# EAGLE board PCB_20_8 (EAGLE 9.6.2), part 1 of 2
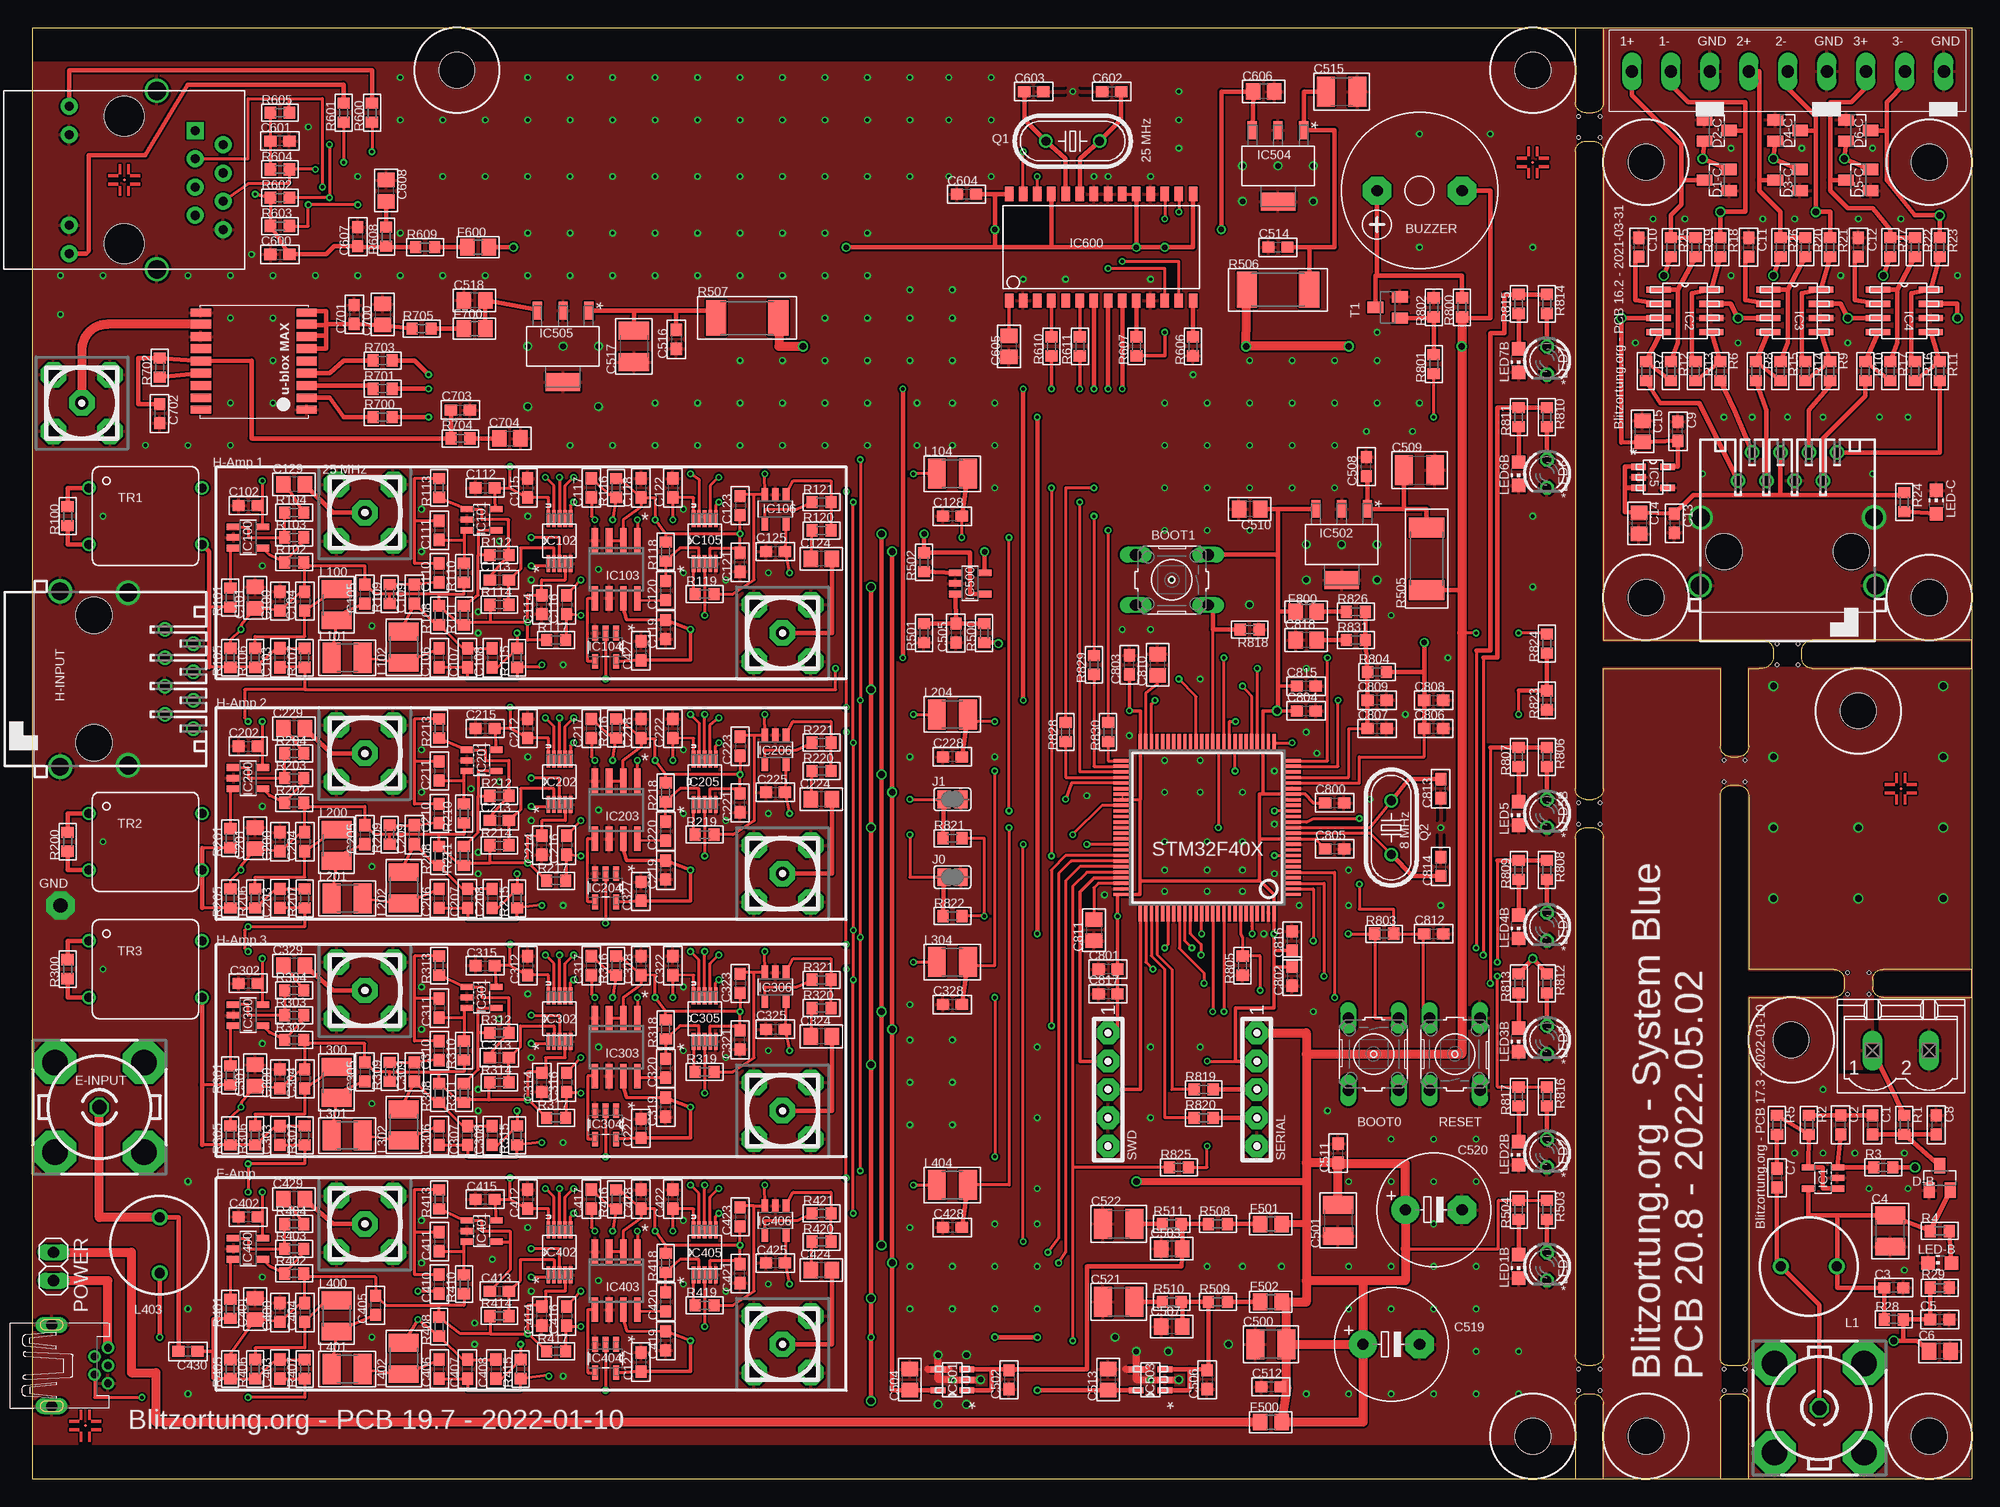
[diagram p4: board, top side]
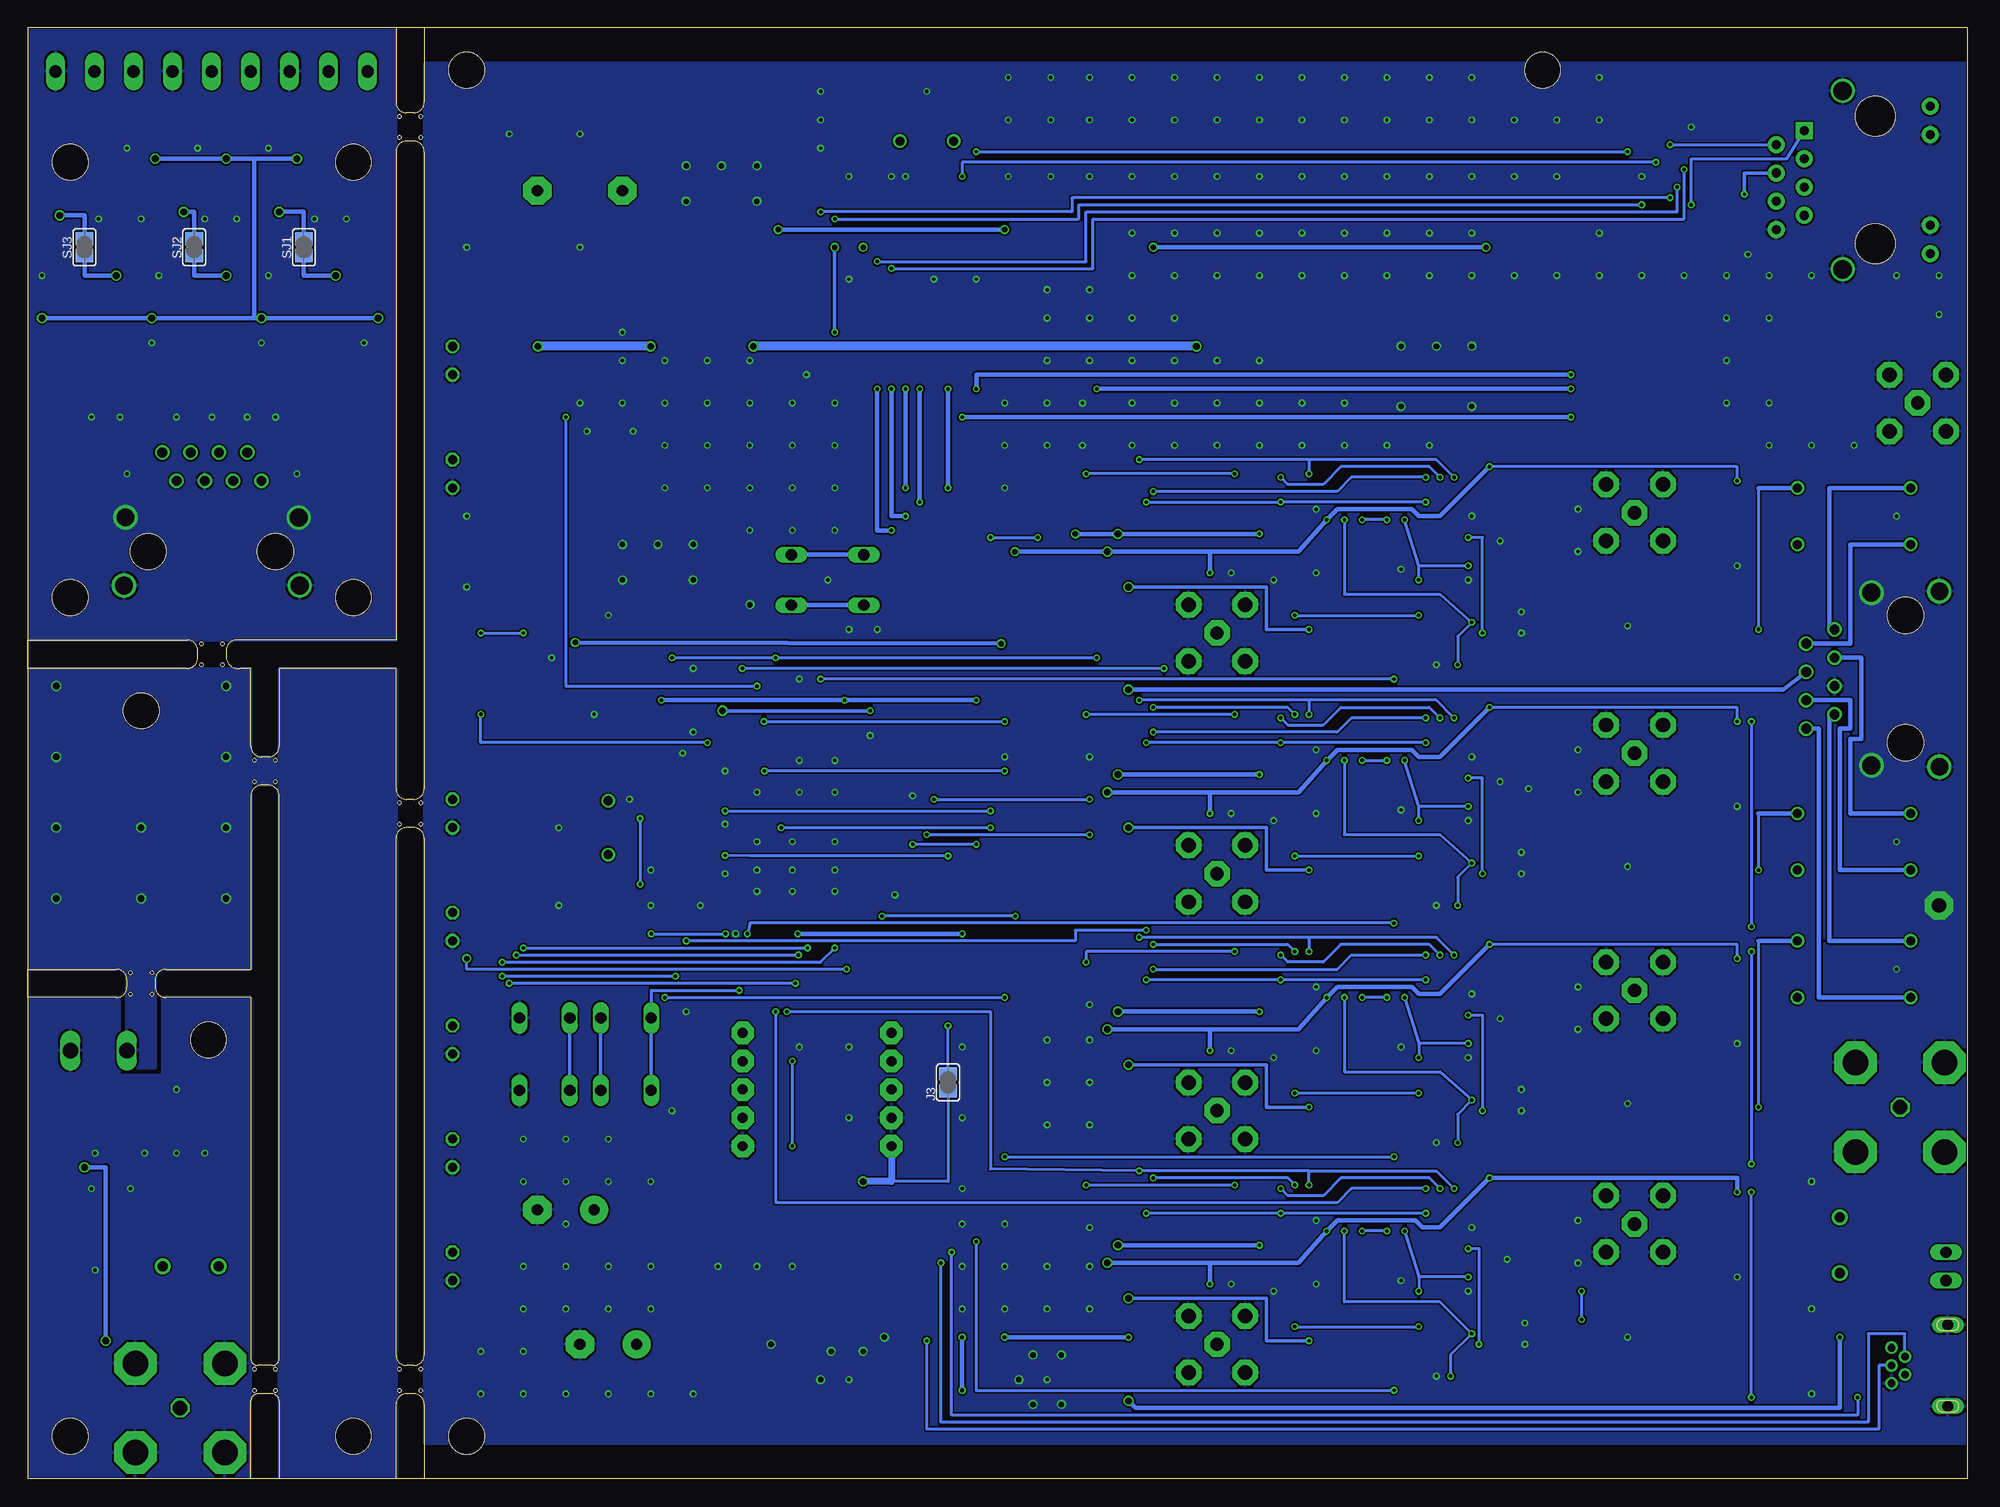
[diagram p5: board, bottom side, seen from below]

Size 173.99 x 130.18 mm. Coordinates in mm from the lower left corner, seen from the top.
Outline: 0,130.18 0,0 173.99,0 173.99,130.18 0,130.18
Copper layers (1*16): Top 0.035mm / dielectric 1.5mm / Bottom 0.035mm
Design rules "default *": minimum track width 6mil, minimum drill 12mil, track to track 6mil, track to pad 6mil, pad to pad 6mil, via to via 6mil, smd to smd 6mil, copper to edge 4mil, drill to drill 8mil, minimum pad ring 8mil, minimum via ring 6mil, stop-mask expansion 3mil, vias tented up to drill 12mil, thermal gap 8mil
Holes 3.2 mm at 134.62,126.36 134.62,3.81 38.1,126.36 157.8,39.37 170.18,3.81 170.18,79.06 144.78,79.06 170.18,118.11 144.78,118.11 163.83,68.9 144.78,3.81
Holes 0.3 mm at 156.53,74.93 158.43,74.93 158.43,73.03 156.53,73.03 138.75,60.64 138.75,58.74 140.65,58.74 140.65,60.64 162.88,43.5 164.78,43.5 164.78,45.4 162.88,45.4 138.75,9.84 138.75,7.94 140.65,7.94 140.65,9.84 151.76,9.84 151.76,7.94 153.67,7.94 153.67,9.84 138.75,122.24 138.75,120.33 140.65,120.33 140.65,122.24 153.67,64.45 151.76,64.45 151.76,62.55 153.67,62.55
tRestrict: 16 lines
Milling: 72 lines

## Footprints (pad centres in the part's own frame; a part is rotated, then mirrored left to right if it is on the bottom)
B3F-10XX = drill 1.016 long: 1 -3.251,2.261; 2 3.251,2.261; 3 -3.251,-2.261; 4 3.251,-2.261
F/CM12P = drill 1.016 pad 2.54 octagon: + 3.81,0; - -3.81,0
C0603 = smd 1.1 x 1: 1 -0.85,0; 2 0.85,0
C1210 = smd 1.6 x 2.7: 1 -1.4,0; 2 1.4,0
C0805 = smd 1.3 x 1.5: 1 -0.95,0; 2 0.95,0
E5-10,5 = drill 1.016 pad 2.54: + -2.54,0 | drill 1.016 pad 2.54 octagon: - 2.54,0
SOT23 = smd 1 x 1.4: 1 -0.95,-1.1; 2 0.95,-1.1; 3 0,1.1
R141426 = drill 1.3 octagon: 1 0,0 | drill 2.286 pad 3.81 octagon: 2 4.008,4.008; 3 -4.008,4.008; 4 -4.008,-4.008; 5 4.008,-4.008
R0805 = smd 1.3 x 1.5: 1 -0.95,0; 2 0.95,0
XLEMO02N = drill 1.3 pad 2.286 octagon: GND@1 -2.54,-2.54; GND@2 2.54,-2.54; GND@3 2.54,2.54; GND@4 -2.54,2.54 | drill 1.2 pad 2.286 octagon: SIG 0,0
556591-1 = drill 0.889: 1 -4.445,6.35; 2 -3.175,8.89; 3 -1.905,6.35; 4 -0.635,8.89; 5 0.635,6.35; 6 1.905,8.89; 7 3.175,6.35; 8 4.445,8.89 | drill 1.575 pad 2.184: G1 -7.874,-3.048; G2 7.874,-3.048 | hole 3.251: -5.715,0; 5.715,0
SOT23-5 = smd 0.55 x 1.2: 1 -0.95,-1.3; 2 0,-1.3; 3 0.95,-1.3; 4 0.95,1.3; 5 -0.95,1.3
SOIC127P600X175-8N = smd 2.184 x 0.559: 1 -2.362,1.905; 2 -2.362,0.635; 3 -2.362,-0.635; 4 -2.362,-1.905; 5 2.362,-1.905; 6 2.362,-0.635; 7 2.362,0.635; 8 2.362,1.905
SOT95P280X110-5N = smd 1.321 x 0.559: 1 -1.295,0.94; 2 -1.295,0; 3 -1.295,-0.94; 4 1.295,-0.94; 5 1.295,0.94
SOT23-5' = smd 0.6 x 1.2: 1 -0.95,-1.306; 2 0,-1.306; 3 0.95,-1.306; 4 0.95,1.306; 5 -0.95,1.306
SOP50P490X110-10N = smd 1.524 x 0.33: 1 -2.032,0.991; 2 -2.032,0.508; 3 -2.032,0; 4 -2.032,-0.508; 5 -2.032,-0.991; 6 2.032,-0.991; 7 2.032,-0.508; 8 2.032,0; 9 2.032,0.508; 10 2.032,0.991
SOIC8 = smd 0.6 x 2.2: 1 -1.905,-2.6; 2 -0.635,-2.6; 3 0.635,-2.6; 4 1.905,-2.6; 5 1.905,2.6; 6 0.635,2.6; 7 -0.635,2.6; 8 -1.905,2.6
SOT95P275X110-5N = smd 1.321 x 0.559: 1 -1.27,0.94; 2 -1.27,0; 3 -1.27,-0.94; 4 1.27,-0.94; 5 1.27,0.94
SOT230P696X180-4N = smd 1.6 x 0.838: 1 -3.2,2.311; 2 -3.2,0; 3 -3.2,-2.311 | smd 1.6 x 3.099: 4 3.2,0
SO28W = smd 0.762 x 1.27: 1 -7.62,-4.78; 2 -6.35,-4.78; 3 -5.08,-4.78; 4 -3.81,-4.78; 5 -2.54,-4.78; 6 -1.27,-4.78; 7 0,-4.78; 8 1.27,-4.78; 9 2.54,-4.78; 10 3.81,-4.78; 11 5.08,-4.78; 12 6.35,-4.78; 13 7.62,-4.78; 14 8.89,-4.78; 15 8.89,4.78; 16 7.62,4.78; 17 6.35,4.78; 18 5.08,4.78; 19 3.81,4.78; 20 2.54,4.78; 21 1.27,4.78; 22 0,4.78; 23 -1.27,4.78; 24 -2.54,4.78; 25 -3.81,4.78; 26 -5.08,4.78; 27 -6.35,4.78; 28 -7.62,4.78
LQFP100 = smd 1.6 x 0.3: 1 -7.6,6; 2 -7.6,5.5; 3 -7.6,5; 4 -7.6,4.5; 5 -7.6,4; 6 -7.6,3.5; 7 -7.6,3; 8 -7.6,2.5; 9 -7.6,2; 10 -7.6,1.5; 11 -7.6,1; 12 -7.6,0.5; 13 -7.6,0; 14 -7.6,-0.5; 15 -7.6,-1; 16 -7.6,-1.5; 17 -7.6,-2; 18 -7.6,-2.5; 19 -7.6,-3; 20 -7.6,-3.5; 21 -7.6,-4; 22 -7.6,-4.5; 23 -7.6,-5; 24 -7.6,-5.5; 25 -7.6,-6; 51 7.6,-6; 52 7.6,-5.5; 53 7.6,-5; 54 7.6,-4.5; 55 7.6,-4; 56 7.6,-3.5; 57 7.6,-3; 58 7.6,-2.5; 59 7.6,-2; 60 7.6,-1.5; 61 7.6,-1; 62 7.6,-0.5; 63 7.6,0; 64 7.6,0.5; 65 7.6,1; 66 7.6,1.5; 67 7.6,2; 68 7.6,2.5; 69 7.6,3; 70 7.6,3.5; 71 7.6,4; 72 7.6,4.5; 73 7.6,5; 74 7.6,5.5; 75 7.6,6 | smd 0.3 x 1.6: 26 -6,-7.6; 27 -5.5,-7.6; 28 -5,-7.6; 29 -4.5,-7.6; 30 -4,-7.6; 31 -3.5,-7.6; 32 -3,-7.6; 33 -2.5,-7.6; 34 -2,-7.6; 35 -1.5,-7.6; 36 -1,-7.6; 37 -0.5,-7.6; 38 0,-7.6; 39 0.5,-7.6; 40 1,-7.6; 41 1.5,-7.6; 42 2,-7.6; 43 2.5,-7.6; 44 3,-7.6; 45 3.5,-7.6; 46 4,-7.6; 47 4.5,-7.6; 48 5,-7.6; 49 5.5,-7.6; 50 6,-7.6; 76 6,7.6; 77 5.5,7.6; 78 5,7.6; 79 4.5,7.6; 80 4,7.6; 81 3.5,7.6; 82 3,7.6; 83 2.5,7.6; 84 2,7.6; 85 1.5,7.6; 86 1,7.6; 87 0.5,7.6; 88 0,7.6; 89 -0.5,7.6; 90 -1,7.6; 91 -1.5,7.6; 92 -2,7.6; 93 -2.5,7.6; 94 -3,7.6; 95 -3.5,7.6; 96 -4,7.6; 97 -4.5,7.6; 98 -5,7.6; 99 -5.5,7.6; 100 -6,7.6
MSTBV2 = drill 1.397 long: 1 -2.54,0; 2 2.54,0
SJ = smd 1.168 x 1.6: 1 -0.762,0; 2 0.762,0
6000-XXXX-RC = drill 0.9 pad 1.422: 1 -2.5,0; 2 2.5,0
R1210 = smd 1.6 x 2.7: 1 -1.4,0; 2 1.4,0
LED3MM = drill 0.813 octagon: A -1.27,0; K 1.27,0
CHIP-LED0805 = smd 1.2 x 1.2: A 0,-1.05; C 0,1.05
PASSER-SMD = smd 0.254 x 0.254: PASS@1 0,0
1X02 = drill 1.016 long: 1 -1.27,0; 2 1.27,0
HC49U-V = drill 0.813: 1 -2.413,0; 2 2.413,0
R0603 = smd 1 x 1.1: 1 -0.85,0; 2 0.85,0
R2512 = smd 1.8 x 3.2: 1 -2.8,0; 2 2.8,0
HR911105A = drill 0.813 pad 1.524: G+ 4.953,-6.604; G- 4.953,-4.064; GND -8.89,4.445; NC -6.35,3.175; P4 -8.89,-0.635; P5 -6.35,0.635; RD+ -6.35,-1.905; RD- -8.89,1.905; TD- -8.89,-3.175; Y+ 4.953,6.604; Y- 4.953,4.064 | drill 1.651 pad 2.159: SHIELD0 -2.921,8.001; SHIELD1 -2.921,-8.001 | drill 0.813 pad 1.524 square: TD+ -6.35,-4.445 | hole 3.556: 0,-5.715; 0,5.715
X05N-SIL = drill 0.889 pad 2.032 octagon: 1 -5.08,0; 2 -2.54,0; 3 0,0; 4 2.54,0; 5 5.08,0
786-4 = drill 0.8: 1 -5.08,2.54; 3 -5.08,-2.54; 4 5.08,-2.54; 6 5.08,2.54
MAX-M8 = smd 1.8 x 0.7: 1_GND 4.95,-4.4; 9_RESET_N 4.95,4.3; 10_GND -4.55,4.3; 18_SAFEBOOT_N -4.55,-4.4 | smd 1.8 x 0.8: 2_TXD 4.95,-3.35; 3_RXD 4.95,-2.25; 4_TIMEPULSE 4.95,-1.15; 5_EXTINT 4.95,-0.05; 6_V_BCKP 4.95,1.05; 7_VCC_IO 4.95,2.15; 8_VCC 4.95,3.25; 11_RF_IN -4.55,3.25; 12_GND -4.55,2.15; 13_LNA_EN -4.55,1.05; 14_VCC_RF -4.55,-0.05; 15_V_ANT/RESERVED -4.55,-1.15; 16_SDA -4.55,-2.25; 17_SCL -4.55,-3.35
32005-601 = drill 0.7 pad 1.016: 1 2.825,1.6; 2 1.625,0.8; 3 2.825,0; 4 1.625,-0.8; 5 2.825,-1.6 | drill 1 pad 1.422 long: M1 -2.225,3.65; M2 -2.225,-3.65
1751316 = drill 1.1 pad 1.7 long: 1 -13.973,-0.1; 2 -10.473,-0.1; 3 -6.973,-0.1; 4 -3.473,-0.1; 5 0.028,-0.1; 6 3.527,-0.1; 7 7.027,-0.1; 8 10.527,-0.1; 9 14.027,-0.1

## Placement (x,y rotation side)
BOOT0  boot0  [B3F-10XX]  120.33,38.1 270 top
BOOT1  boot1  [B3F-10XX]  102.23,80.64 180 top
BUZZER  F/CM12P  [F/CM12P]  124.46,115.57 180 top
C1  10pF  [C0603]  165.1,31.75 270 top
C2  10pF  [C0603]  162.24,31.75 90 top
C3  1uF  [C0603]  167,17.14 180 top
C4  47uF  [C1210]  166.69,22.23 90 top
C5  1uF  [C0603]  171.13,14.29 180 top
C6  10uF  [C0805]  171.13,11.43 180 top
C7  1uF  [C0603]  156.53,26.99 90 top
C8  47pF  [C0603]  170.81,31.75 270 top
C9  100nF  [C0603]  147.64,93.98 90 top
C10  100nF  [C0603]  144.15,110.49 90 top
C11  100nF  [C0603]  153.99,110.49 90 top
C12  100nF  [C0603]  163.83,110.49 90 top
C13  100nF  [C0603]  147.32,85.72 270 top
C14  10uF  [C0805]  144.15,85.72 270 top
C15  10uF  [C0805]  144.46,93.98 90 top
C100  1uF  [C0603]  22.23,78.74 270 top
C101  10uF  [C0805]  20,79.06 270 top
C102  1uF  [C0603]  19.37,87.31 0 top
C103  4.7pF  [C0603]  22.23,73.66 90 top
C104  1.5nF  [C0603]  24.45,78.74 270 top
C105  6.8nF  [C0603]  29.84,79.38 270 top
C106  12nF  [C0603]  36.51,73.66 90 top
C107  22nF  [C0603]  39.05,73.66 90 top
C108  2.2nF  [C0603]  41.27,73.66 270 top
C109  1nF  [C0603]  34.29,79.38 90 top
C110  1nF  [C0603]  36.51,81.28 90 top
C111  1nF  [C0603]  36.51,85.09 270 top
C112  1uF  [C0603]  40.64,88.9 0 top
C113  1uF  [C0603]  41.91,80.64 0 top
C114  1uF  [C0603]  45.72,78.42 90 top
C115  1uF  [C0603]  44.45,88.9 270 top
C116  1uF  [C0603]  47.94,78.42 270 top
C117  1uF  [C0603]  50.16,88.9 90 top
C118  1uF  [C0603]  54.61,88.9 270 top
C119  1uF  [C0603]  56.83,76.2 90 top
C120  1uF  [C0603]  56.83,79.69 90 top
C121  1uF  [C0603]  63.5,82.23 90 top
C122  1uF  [C0603]  57.47,88.9 270 top
C123  750pF  [C0603]  63.5,87.31 270 top
C124  10uF  [C0805]  70.8,82.55 180 top
C125  1uF  [C0603]  66.67,83.19 0 top
C127  100nF  [C0603]  54.61,10.48 270 top
C128  3.3nF  [C0603]  82.55,86.36 180 top
C129  10uF  [C0805]  23.5,89.22 180 top
C200  1uF  [C0603]  22.23,57.15 270 top
C201  10uF  [C0805]  20,57.47 270 top
C202  1uF  [C0603]  19.37,65.72 0 top
C203  4.7pF  [C0603]  22.23,52.07 90 top
C204  1.5nF  [C0603]  24.45,57.15 270 top
C205  6.8nF  [C0603]  29.84,57.78 270 top
C206  12nF  [C0603]  36.51,52.07 90 top
C207  22nF  [C0603]  39.05,52.07 90 top
C208  2.2nF  [C0603]  41.27,52.07 270 top
C209  1nF  [C0603]  34.29,57.78 90 top
C210  1nF  [C0603]  36.51,59.69 90 top
C211  1nF  [C0603]  36.51,63.5 270 top
C212  1uF  [C0603]  44.45,67.31 270 top
C213  1uF  [C0603]  41.91,59.05 0 top
C214  1uF  [C0603]  45.72,56.83 90 top
C215  1uF  [C0603]  40.64,67.31 0 top
C216  1uF  [C0603]  47.94,56.83 270 top
C217  1uF  [C0603]  50.16,67.31 90 top
C218  1uF  [C0603]  54.61,67.31 270 top
C219  1uF  [C0603]  56.83,54.61 90 top
C220  1uF  [C0603]  56.83,58.1 90 top
C221  1uF  [C0603]  63.5,60.64 90 top
C222  1uF  [C0603]  57.47,67.31 270 top
C223  750pF  [C0603]  63.5,65.72 270 top
C224  10uF  [C0805]  70.8,60.96 180 top
C225  1uF  [C0603]  66.67,61.59 0 top
C227  100nF  [C0603]  54.61,31.43 270 top
C228  3.3nF  [C0603]  82.55,64.77 180 top
C229  10uF  [C0805]  23.5,67.31 180 top
C300  1uF  [C0603]  22.23,35.88 270 top
C301  10uF  [C0805]  20,36.2 270 top
C302  1uF  [C0603]  19.37,44.45 0 top
C303  4.7pF  [C0603]  22.23,30.8 90 top
C304  1.5nF  [C0603]  24.45,35.88 270 top
C305  6.8nF  [C0603]  29.84,36.51 270 top
C306  12nF  [C0603]  36.51,30.8 90 top
C307  22nF  [C0603]  39.05,30.8 90 top
C308  2.2nF  [C0603]  41.27,30.8 270 top
C309  1nF  [C0603]  34.29,36.51 90 top
C310  1nF  [C0603]  36.51,38.42 90 top
C311  1nF  [C0603]  36.51,42.23 270 top
C312  1uF  [C0603]  44.45,46.04 270 top
C313  1uF  [C0603]  41.91,37.78 0 top
C314  1uF  [C0603]  45.72,35.56 90 top
C315  1uF  [C0603]  40.64,46.04 0 top
C316  1uF  [C0603]  47.94,35.56 270 top
C317  1uF  [C0603]  50.16,46.04 90 top
C318  1uF  [C0603]  54.61,46.04 270 top
C319  1uF  [C0603]  56.83,33.34 90 top
C320  1uF  [C0603]  56.83,36.83 90 top
C321  1uF  [C0603]  63.5,39.37 90 top
C322  1uF  [C0603]  57.47,46.04 270 top
C323  750pF  [C0603]  63.5,44.45 270 top
C324  10uF  [C0805]  70.8,39.69 180 top
C325  1uF  [C0603]  66.67,40.32 0 top
C327  100nF  [C0603]  54.61,52.7 270 top
C328  3.3nF  [C0603]  82.55,42.55 180 top
C329  10uF  [C0805]  23.5,46.04 180 top
C400  1uF  [C0603]  22.23,14.92 270 top
C401  10uF  [C0805]  20,15.24 270 top
C402  1uF  [C0603]  19.37,23.5 0 top
C403  4.7pF  [C0603]  22.23,9.84 90 top
C404  1.5nF  [C0603]  24.45,14.92 270 top
C405  6.8nF  [C0603]  30.8,15.56 270 top
C406  12nF  [C0603]  36.51,9.84 90 top
C407  22nF  [C0603]  39.05,9.84 90 top
C408  2.2nF  [C0603]  41.59,9.84 270 top
C410  1nF  [C0603]  36.51,17.46 90 top
C411  1nF  [C0603]  36.51,21.27 270 top
C412  1uF  [C0603]  44.45,25.08 270 top
C413  1uF  [C0603]  41.91,16.83 0 top
C414  1uF  [C0603]  45.72,14.61 90 top
C415  1uF  [C0603]  40.64,25.08 0 top
C416  1uF  [C0603]  47.94,14.61 270 top
C417  1uF  [C0603]  50.16,25.08 90 top
C418  1uF  [C0603]  54.61,25.08 270 top
C419  1uF  [C0603]  56.83,12.38 90 top
C420  1uF  [C0603]  56.83,15.88 90 top
C421  1uF  [C0603]  63.5,18.41 90 top
C422  1uF  [C0603]  57.47,25.08 270 top
C423  750pF  [C0603]  63.5,23.5 270 top
C424  10uF  [C0805]  70.8,18.73 180 top
C425  1uF  [C0603]  66.67,19.37 0 top
C427  100nF  [C0603]  54.61,74.3 270 top
C428  3.3nF  [C0603]  82.55,22.54 180 top
C429  10uF  [C0805]  23.5,25.08 180 top
C430  1uF  [C0603]  13.97,11.43 0 top
C500  47uF  [C1210]  111.12,12.06 180 top
C501  47uF  [C1210]  117.16,23.18 270 top
C502  100nF  [C0603]  87.63,8.89 270 top
C503  10uF  [C0805]  102.23,20.64 180 top
C504  10uF  [C0805]  78.74,8.89 90 top
C505  1uF  [C0603]  82.87,75.88 270 top
C506  100nF  [C0603]  105.41,8.89 270 top
C507  10uF  [C0805]  102.23,13.65 180 top
C508  100nF  [C0603]  119.7,90.81 90 top
C509  47uF  [C1210]  124.46,90.49 0 top
C510  10uF  [C0805]  109.22,87 180 top
C511  100nF  [C0603]  117.16,29.21 90 top
C512  100nF  [C0603]  111.12,8.26 180 top
C513  10uF  [C0805]  96.52,8.89 90 top
C514  100nF  [C0603]  111.76,110.49 180 top
C515  47uF  [C1210]  117.47,124.46 0 top
C516  100nF  [C0603]  57.78,102.23 270 top
C517  47uF  [C1210]  53.98,101.6 270 top
C518  10uF  [C0805]  39.69,105.73 180 top
C519  1000uF  [E5-10,5]  121.92,12.06 0 top
C520  1000uF  [E5-10,5]  125.73,24.13 0 top
C521  47uF  [C1210]  97.47,15.88 0 top
C522  47uF  [C1210]  97.47,22.86 0 top
C600  100nF  [C0603]  22.23,109.86 0 top
C601  100nF  [C0603]  22.23,120.02 180 top
C602  18pF  [C0603]  96.84,124.46 0 top
C603  18pF  [C0603]  89.85,124.46 180 top
C604  100nF  [C0603]  83.82,115.25 0 top
C605  10uF  [C0805]  87.63,101.6 90 top
C606  10uF  [C0805]  110.49,124.46 180 top
C607  1uF  [C0603]  29.21,111.44 90 top
C608  10uF  [C0805]  31.75,115.57 90 top
C700  10uF  [C0805]  31.43,104.46 270 top
C701  100nF  [C0603]  28.89,104.46 270 top
C702  100nF  [C0603]  11.43,95.57 270 top
C703  1uF  [C0603]  38.42,95.89 0 top
C704  10uF  [C0805]  42.86,93.34 0 top
C800  100nF  [C0603]  116.84,60.64 0 top
C801  100nF  [C0603]  96.52,45.72 180 top
C802  100nF  [C0603]  113.03,45.09 270 top
C803  100nF  [C0603]  98.42,73.03 90 top
C804  100nF  [C0603]  114.3,68.9 0 top
C805  100nF  [C0603]  116.84,56.52 0 top
C806  1uF  [C0603]  125.73,67.31 0 top
C807  1uF  [C0603]  120.65,67.31 180 top
C808  100nF  [C0603]  125.73,69.85 0 top
C809  100nF  [C0603]  120.65,69.85 180 top
C810  10uF  [C0805]  100.97,73.03 90 top
C811  10uF  [C0805]  95.25,49.21 270 top
C812  100nF  [C0603]  125.73,48.9 0 top
C813  18pF  [C0603]  126.36,61.91 90 top
C814  18pF  [C0603]  126.36,54.93 270 top
C815  1uF  [C0603]  114.3,71.12 0 top
C816  1uF  [C0603]  113.03,48.26 90 top
C817  1uF  [C0603]  96.52,43.5 180 top
C818  10uF  [C0805]  114.3,75.25 180 top
D1-C  BAT54S  [SOT23]  151.13,116.52 90 top
D2-C  BAT54S  [SOT23]  151.13,120.97 270 top
D3-C  BAT54S  [SOT23]  157.48,116.52 90 top
D4-C  BAT54S  [SOT23]  157.48,120.97 270 top
D5-C  BAT54S  [SOT23]  163.83,116.52 90 top
D6-C  BAT54S  [SOT23]  163.83,120.97 270 top
D-B  BAT54S  [SOT23]  171.13,26.99 0 top
E-INPUT  [R141426]  6.03,33.34 0 top
F500  60  [R0805]  111.12,5.08 180 top
F501  220  [R0805]  111.12,22.86 180 top
F502  220  [R0805]  111.12,15.88 180 top
F600  60  [R0805]  40.01,110.49 180 top
F700  60  [R0805]  39.69,103.19 180 top
F800  220  [R0805]  114.3,77.79 180 top
GPS-IN  GPS-IN  [XLEMO02N]  4.45,96.52 0 top
H-INPUT  RJ45  [556591-1]  5.56,71.75 270 top
IC1  ADA4891  [SOT23-5]  160.66,26.99 90 top
IC2  THS4531ID  [SOIC127P600X175-8N]  148.27,104.78 0 top
IC3  THS4531ID  [SOIC127P600X175-8N]  158.12,104.78 0 top
IC4  THS4531ID  [SOIC127P600X175-8N]  167.96,104.78 0 top
IC5  TLV70033  [SOT95P280X110-5N]  145.41,89.85 0 top
IC100  MCP6021  [SOT23-5']  19.37,84.45 270 top
IC101  ADA4891  [SOT23-5]  40.32,86.04 270 top
IC102  MCP6S93-E/UN  [SOP50P490X110-10N]  47.31,84.14 90 top
IC103  LTC1569CS8-7  [SOIC8]  52.39,81.6 180 top
IC104  MC74HC1G04DTT1G  [SOT95P275X110-5N]  51.44,74.61 270 top
IC105  MCP6S93-E/UN  [SOP50P490X110-10N]  60.33,84.14 90 top
IC106  MCP6021  [SOT23-5']  66.67,87 180 top
IC200  MCP6021  [SOT23-5']  19.37,62.87 270 top
IC201  ADA4891  [SOT23-5]  40.32,64.45 270 top
IC202  MCP6S93-E/UN  [SOP50P490X110-10N]  47.31,62.55 90 top
IC203  LTC1569CS8-7  [SOIC8]  52.39,60.01 180 top
IC204  MC74HC1G04DTT1G  [SOT95P275X110-5N]  51.44,53.02 270 top
IC205  MCP6S93-E/UN  [SOP50P490X110-10N]  60.33,62.55 90 top
IC206  MCP6021  [SOT23-5']  66.67,65.41 180 top
IC300  MCP6021  [SOT23-5']  19.37,41.59 270 top
IC301  ADA4891  [SOT23-5]  40.32,43.18 270 top
IC302  MCP6S93-E/UN  [SOP50P490X110-10N]  47.31,41.27 90 top
IC303  LTC1569CS8-7  [SOIC8]  52.39,38.73 180 top
IC304  MC74HC1G04DTT1G  [SOT95P275X110-5N]  51.44,31.75 270 top
IC305  MCP6S93-E/UN  [SOP50P490X110-10N]  60.33,41.27 90 top
IC306  MCP6021  [SOT23-5']  66.67,44.13 180 top
IC400  MCP6021  [SOT23-5']  19.37,20.64 270 top
IC401  ADA4891  [SOT23-5]  40.32,22.23 270 top
IC402  MCP6S93-E/UN  [SOP50P490X110-10N]  47.31,20.32 90 top
IC403  LTC1569CS8-7  [SOIC8]  52.39,17.78 180 top
IC404  MC74HC1G04DTT1G  [SOT95P275X110-5N]  51.44,10.79 270 top
IC405  MCP6S93-E/UN  [SOP50P490X110-10N]  60.33,20.32 90 top
IC406  MCP6021  [SOT23-5']  66.67,23.18 180 top
IC500  ADA4891  [SOT23-5']  84.14,80.33 270 top
IC501  TLV70033  [SOT95P280X110-5N]  82.55,8.89 180 top
IC502  LM3940IMP-3.3  [SOT230P696X180-4N]  117.47,83.82 270 top
IC503  LP5907MFX-4.5NPB  [SOT95P280X110-5N]  100.33,8.89 180 top
IC504  LM3940IMP-3.3  [SOT230P696X180-4N]  111.76,117.79 270 top
IC505  LM3940IMP-3.3  [SOT230P696X180-4N]  47.62,101.6 270 top
IC600  ENC28J60SO  [SO28W]  95.25,110.49 0 top
IC800  STM32D40X  [LQFP100]  105.41,58.42 180 top
IN  MSTBV2  [MSTBV2]  167.64,38.42 0 top
J0  J0  [SJ]  82.55,53.98 0 top
J1  J1  [SJ]  82.55,60.96 0 top
J2  Amplifier  [556591-1]  157.48,83.19 0 top
J3  J1  [SJ]  91.44,35.56 90 bottom
L1  3.3mH  [6000-XXXX-RC]  159.38,19.05 180 top
L100  330uH  [R1210]  27.3,78.42 270 top
L101  680uH  [R1210]  28.26,73.66 0 top
L102  1mH  [R1210]  33.34,74.61 90 top
L104  22uH  [R1210]  82.55,90.17 180 top
L200  330uH  [R1210]  27.3,56.83 270 top
L201  680uH  [R1210]  28.26,52.07 0 top
L202  1mH  [R1210]  33.34,53.02 90 top
L204  22uH  [R1210]  82.55,68.58 180 top
L300  330uH  [R1210]  27.3,35.56 270 top
L301  680uH  [R1210]  28.26,30.8 0 top
L302  1mH  [R1210]  33.34,31.75 90 top
L304  22uH  [R1210]  82.55,46.35 180 top
L400  330uH  [R1210]  27.3,14.61 270 top
L401  680uH  [R1210]  28.26,9.84 0 top
L402  1mH  [R1210]  33.34,10.79 90 top
L403  3.3mH  [6000-XXXX-RC]  11.43,20.95 90 top
L404  22uH  [R1210]  82.55,26.35 180 top
LED1  Power  [LED3MM]  135.89,19.05 270 top
LED1B  Power  [CHIP-LED0805]  133.35,19.05 180 top
LED2  Mode  [LED3MM]  135.89,29.21 270 top
LED2B  Mode  [CHIP-LED0805]  133.35,29.21 180 top
LED3  Network  [LED3MM]  135.89,39.37 270 top
LED3B  Network  [CHIP-LED0805]  133.35,39.37 180 top
LED4  Fault  [LED3MM]  135.89,49.53 270 top
LED4B  Fault  [CHIP-LED0805]  133.35,49.53 180 top
LED5  GPS  [LED3MM]  135.89,59.69 270 top
LED5B  GPS  [CHIP-LED0805]  133.35,59.69 180 top
LED6  Alarm  [LED3MM]  135.89,90.17 270 top
LED6B  Alarm  [CHIP-LED0805]  133.35,90.17 180 top
LED7  Signal  [LED3MM]  135.89,100.33 270 top
LED7B  Signal  [CHIP-LED0805]  133.35,100.33 180 top
LED-B  LED-B  [CHIP-LED0805]  171.13,19.37 90 top
LED-C  LED-C  [CHIP-LED0805]  170.81,87.63 0 top
OUT  R141426  [R141426]  160.34,6.35 270 top
PASSER1  [PASSER-SMD]  4.76,4.76 0 top
PASSER2  [PASSER-SMD]  8.26,116.52 0 top
PASSER3  [PASSER-SMD]  134.62,118.11 0 top
PASSER4  [PASSER-SMD]  167.64,61.91 0 top
POWER  power  [1X02]  1.91,19.05 270 top
Q1  25MHz  [HC49U-V]  93.34,120.02 0 top
Q2  8MHz  [HC49U-V]  121.92,58.42 90 top
R1  10K  [R0603]  167.96,31.75 90 top
R2  5.6M  [R0603]  159.38,31.75 90 top
R3  10M  [R0603]  166.05,27.94 180 top
R4  2.2K  [R0603]  171.13,22.23 180 top
R5  75  [R0603]  156.53,31.75 270 top
R6  49.9  [R0603]  151.45,99.38 270 top
R7  49.9  [R0603]  144.78,99.38 270 top
R8  49.9  [R0603]  154.62,99.38 270 top
R9  49.9  [R0603]  161.29,99.38 270 top
R10  49.9  [R0603]  164.47,99.38 270 top
R11  49.9  [R0603]  171.13,99.38 270 top
R12  10K  [R0603]  147,99.38 90 top
R13  10K  [R0603]  149.22,99.38 90 top
R14  10K  [R0603]  159.07,99.38 90 top
R15  10K  [R0603]  156.84,99.38 90 top
R16  10K  [R0603]  168.91,99.38 90 top
R17  10K  [R0603]  166.69,99.38 90 top
R18  1K  [R0603]  151.45,110.49 90 top
R19  1K  [R0603]  149.22,110.49 90 top
R20  1K  [R0603]  159.07,110.49 90 top
R21  1K  [R0603]  161.29,110.49 90 top
R22  1K  [R0603]  168.91,110.49 90 top
R23  1K  [R0603]  171.13,110.49 90 top
R24  2.2K  [R0603]  167.96,87.63 270 top
R25  160  [R0603]  147,110.49 270 top
R26  160  [R0603]  156.84,110.49 270 top
R27  160  [R0603]  166.69,110.49 270 top
R28  100K  [R0603]  167,14.29 180 top
R29  100K  [R0603]  171.13,17.14 180 top
R100  160  [R0603]  3.17,86.36 90 top
R101  1K  [R0603]  17.78,79.06 90 top
R102  1K  [R0603]  23.5,82.23 0 top
R103  1K  [R0603]  23.5,84.45 0 top
R104  49.9  [R0603]  23.5,86.68 0 top
R105  330  [R0603]  17.78,73.66 270 top
R106  270  [R0603]  20,73.66 90 top
R107  47K  [R0603]  24.45,73.66 270 top
R108  2.2K  [R0603]  36.51,77.47 270 top
R109  51K  [R0603]  32.07,79.38 90 top
R110  100K  [R0603]  38.73,81.28 90 top
R111  10K  [R0603]  38.73,77.47 90 top
R112  30K  [R0603]  41.91,82.87 0 top
R113  200K  [R0603]  36.51,88.9 270 top
R114  10K  [R0603]  41.91,78.42 0 top
R115  22K  [R0603]  43.5,73.66 90 top
R116  10K  [R0603]  52.39,88.9 270 top
R117  10K  [R0603]  46.99,75.25 0 top
R118  10K  [R0603]  56.83,83.19 270 top
R119  100  [R0603]  60.33,79.38 0 top
R120  49.9  [R0603]  70.8,85.09 180 top
R121  1K  [R0603]  70.8,87.63 0 top
R200  160  [R0603]  3.17,57.15 90 top
R201  1K  [R0603]  17.78,57.47 90 top
R202  1K  [R0603]  23.5,60.64 0 top
R203  1K  [R0603]  23.5,62.87 0 top
R204  49.9  [R0603]  23.5,65.09 0 top
R205  330  [R0603]  17.78,52.07 270 top
R206  270  [R0603]  20,52.07 90 top
R207  47K  [R0603]  24.45,52.07 270 top
R208  2.2K  [R0603]  36.51,55.88 270 top
R209  51K  [R0603]  32.07,57.78 90 top
R210  100K  [R0603]  38.73,59.69 90 top
R211  10K  [R0603]  38.73,55.88 90 top
R212  30K  [R0603]  41.91,61.28 0 top
R213  200K  [R0603]  36.51,67.31 270 top
R214  10K  [R0603]  41.91,56.83 0 top
R215  22K  [R0603]  43.5,52.07 90 top
R216  10K  [R0603]  52.39,67.31 270 top
R217  10K  [R0603]  46.99,53.66 0 top
R218  10K  [R0603]  56.83,61.59 270 top
R219  100  [R0603]  60.33,57.78 0 top
R220  49.9  [R0603]  70.8,63.5 180 top
R221  1K  [R0603]  70.8,66.04 0 top
R300  160  [R0603]  3.17,45.72 90 top
R301  1K  [R0603]  17.78,36.2 90 top
R302  1K  [R0603]  23.5,39.37 0 top
R303  1K  [R0603]  23.5,41.59 0 top
R304  49.9  [R0603]  23.5,43.81 0 top
R305  330  [R0603]  17.78,30.8 270 top
R306  270  [R0603]  20,30.8 90 top
R307  47K  [R0603]  24.45,30.8 270 top
R308  2.2K  [R0603]  36.51,34.61 270 top
R309  51K  [R0603]  32.07,36.51 90 top
R310  100K  [R0603]  38.73,38.42 90 top
R311  10K  [R0603]  38.73,34.61 90 top
R312  30K  [R0603]  41.91,40.01 0 top
R313  200K  [R0603]  36.51,46.04 270 top
R314  10K  [R0603]  41.91,35.56 0 top
R315  22K  [R0603]  43.5,30.8 90 top
R316  10K  [R0603]  52.39,46.04 270 top
R317  10K  [R0603]  46.99,32.38 0 top
R318  10K  [R0603]  56.83,40.32 270 top
R319  100  [R0603]  60.33,36.51 0 top
R320  49.9  [R0603]  70.8,42.23 180 top
R321  1K  [R0603]  70.8,44.77 0 top
R401  1K  [R0603]  17.78,15.24 90 top
R402  1K  [R0603]  23.5,18.41 0 top
R403  1K  [R0603]  23.5,20.64 0 top
R404  49.9  [R0603]  23.5,22.86 0 top
R405  82  [R0603]  17.78,9.84 90 top
R406  270  [R0603]  20,9.84 90 top
R407  47K  [R0603]  24.45,9.84 270 top
R408  2.2K  [R0603]  36.51,13.65 90 top
R410  150K  [R0603]  38.73,17.46 90 top
R413  68K  [R0603]  36.51,25.08 270 top
R414  10K  [R0603]  41.91,14.61 0 top
R415  22K  [R0603]  43.81,9.84 90 top
R416  10K  [R0603]  52.39,25.08 270 top
R417  10K  [R0603]  46.99,11.43 0 top
R418  10K  [R0603]  56.83,19.37 270 top
R419  100  [R0603]  60.33,15.56 0 top
R420  49.9  [R0603]  70.8,21.27 180 top
R421  1K  [R0603]  70.8,23.81 0 top
R500  1M  [R0603]  85.41,75.88 90 top
R501  1M  [R0603]  80.01,75.88 270 top
R502  10  [R0603]  80.01,82.23 270 top
R503  1K  [R0603]  135.89,24.13 90 top
R504  2.2K  [R0603]  133.35,24.13 90 top
R505  1.5  [R2512]  125.09,82.55 90 top
R506  1.5  [R2512]  111.76,106.68 0 top
R507  1.5  [R2512]  64.14,104.14 180 top
R508  0.27  [R0603]  106.36,22.86 180 top
R509  0.27  [R0603]  106.36,15.88 180 top
R510  0.27  [R0603]  102.23,15.88 0 top
R511  0.27  [R0603]  102.23,22.86 0 top
R600  680  [R0603]  30.48,122.56 90 top
R601  680  [R0603]  27.94,122.56 90 top
R602  49.9  [R0603]  22.23,114.94 180 top
R603  49.9  [R0603]  22.23,112.39 180 top
R604  49.9  [R0603]  22.23,117.47 0 top
R605  49.9  [R0603]  22.23,122.56 0 top
R606  2.2K  [R0603]  104.14,101.6 90 top
R607  10K  [R0603]  99.06,101.6 270 top
R608  0.27  [R0603]  31.75,111.44 270 top
R609  0.27  [R0603]  35.24,110.49 180 top
R610  75  [R0603]  91.44,101.6 270 top
R611  75  [R0603]  93.98,101.6 270 top
R700  470  [R0603]  31.43,95.25 180 top
R701  470  [R0603]  31.43,97.79 180 top
R702  10  [R0603]  11.43,99.69 90 top
R703  100  [R0603]  31.43,100.33 180 top
R704  0.27  [R0603]  38.42,93.34 180 top
R705  0.27  [R0603]  34.92,103.19 180 top
R800  470  [R0603]  128.27,105.09 270 top
R801  2.2K  [R0603]  125.73,100.01 270 top
R802  2.2K  [R0603]  125.73,105.09 270 top
R803  2.2K  [R0603]  121.28,48.9 180 top
R804  5.1  [R0603]  120.65,72.39 0 top
R805  10K  [R0603]  108.58,46.04 90 top
R806  4.7K  [R0603]  135.89,64.77 90 top
R807  1K  [R0603]  133.35,64.77 90 top
R808  330  [R0603]  135.89,54.61 90 top
R809  1K  [R0603]  133.35,54.61 90 top
R810  330  [R0603]  135.89,95.25 90 top
R811  1K  [R0603]  133.35,95.25 90 top
R812  330  [R0603]  135.89,44.45 90 top
R813  1K  [R0603]  133.35,44.45 90 top
R814  330  [R0603]  135.89,105.41 90 top
R815  1K  [R0603]  133.35,105.41 90 top
R816  330  [R0603]  135.89,34.29 90 top
R817  1K  [R0603]  133.35,34.29 90 top
R818  2.2K  [R0603]  109.22,76.2 180 top
R819  330  [R0603]  105.09,34.92 0 top
R820  330  [R0603]  105.09,32.38 0 top
R821  100K  [R0603]  82.55,57.47 180 top
R822  100K  [R0603]  82.55,50.48 180 top
R823  10K  [R0603]  135.89,69.85 90 top
R824  10K  [R0603]  135.89,74.93 90 top
R825  1K  [R0603]  102.87,27.94 0 top
R826  0.27  [R0603]  118.75,77.79 180 top
R828  75  [R0603]  92.71,66.99 90 top
R829  75  [R0603]  95.25,73.03 90 top
R830  75  [R0603]  96.52,66.99 90 top
R831  0.27  [R0603]  118.75,75.25 180 top
RESET  reset  [B3F-10XX]  127.64,38.1 90 top
RJ1  HR911105A  [HR911105A]  8.26,116.52 180 top
SERIAL  serial  [X05N-SIL]  109.86,34.92 270 top
SJ1  J1  [SJ]  149.22,110.49 90 bottom
SJ2  J2  [SJ]  159.07,110.49 90 bottom
SJ3  J3  [SJ]  168.91,110.49 90 bottom
SMA10  A  [XLEMO02N]  29.84,86.68 0 top
SMA11  B  [XLEMO02N]  67.31,75.88 0 top
SMA20  A  [XLEMO02N]  29.84,65.09 0 top
SMA21  B  [XLEMO02N]  67.31,54.29 0 top
SMA30  A  [XLEMO02N]  29.84,43.81 0 top
SMA31  B  [XLEMO02N]  67.31,33.02 0 top
SMA40  A  [XLEMO02N]  29.84,22.86 0 top
SMA41  B  [XLEMO02N]  67.31,12.06 0 top
SWD  SWD  [X05N-SIL]  96.52,34.92 270 top
T1  BC847  [SOT23]  121.6,105.09 90 top
TR1  DA103C  [786-4]  10.16,86.36 0 top
TR2  DA103C  [786-4]  10.16,57.15 0 top
TR3  DA103C  [786-4]  10.16,45.72 0 top
U$1  MAX-M8  [MAX-M8]  19.68,100.33 0 top
USB  [32005-601]  3.97,10.16 0 top
X1  Input  [1751316]  157.48,126.36 0 top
